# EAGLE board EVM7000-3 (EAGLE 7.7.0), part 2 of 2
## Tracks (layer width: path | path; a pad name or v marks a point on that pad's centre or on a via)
109
  Top 0.305: IC30.10 58.42,83.19 57.15,81.92 55.24,81.92 54.61,82.55 54.61,88.27 52.7,90.17 JP3.1
175  (via drill 0.5)
  Top 0.305: IC7.9 16.51,93.98 v16.51,78.11
  Bottom 0.305: v16.51,78.11 120.65,78.11 128.27,70.48 151.13,70.48 154.31,67.31 154.31,64.14 152.4,62.23 IC15.23
243  (via drill 0.5)
  Top 0.305: v36.2,130.81 v36.2,79.38
  Bottom 0.305: IC8.1 11.43,134.62 15.24,130.81 v36.2,130.81 | v36.2,79.38 36.83,78.74 121.28,78.74 128.91,71.12 151.76,71.12 154.94,67.94 154.94,62.23 152.4,59.69 IC15.22
6522  (via drill 0.5)
  Top 0.305: v41.27,80.01 41.27,90.17 v42.55,91.44
  Bottom 0.305: v42.55,91.44 IC34.23 | IC15.21 152.4,57.15 155.57,60.33 155.57,68.58 152.4,71.75 129.54,71.75 121.92,79.38 41.91,79.38 v41.27,80.01
!ENABLE  (via drill 0.5)
  Top 0.305: IC1.16 37.47,59.69 35.56,57.78 35.56,46.35 v37.47,44.45 | IC29.19 69.22,44.45 67.31,42.55 v67.31,38.1
  Bottom 0.305: v37.47,44.45 46.99,44.45 48.26,45.72 52.7,45.72 60.33,38.1 v67.31,38.1 67.94,38.1 73.03,33.02 88.9,33.02 90.17,31.75 IC33.3
+12V  (3 unrouted)
  Bottom 1.27: 133.35,9.53 X1.4 132.72,17.78 C26.+ | 154.31,9.53 VR1.1 | 149.22,9.53 144.78,13.34 | P3.3 161.29,35.56 158.12,32.38 151.76,32.38 149.86,30.48 149.86,24.77 C27.1 142.24,17.14 142.24,13.34
  Bottom 2.54: 133.35,9.53 137.16,9.53 137.16,9.87 J3.2 137.79,10.16 140.81,13.18 144.94,13.18 149.22,9.53 154.31,9.53
/LA  (via drill 0.5)
  Top 0.305: IC33.17 101.6,19.05 103.5,20.95 103.5,80.64 v101.6,82.55
  Bottom 0.305: IC30.4 66.04,90.81 68.58,88.27 73.03,88.27 76.2,85.09 99.06,85.09 v101.6,82.55
A0  (via drill 0.5)
  Top 0.305: IC21.12 93.98,44.45 97.16,47.62 97.16,78.74 98.42,80.01 v98.42,81.92 | IC34.37 47.62,127 44.45,123.83 44.45,83.19 43.81,82.55 v43.81,81.28
  Bottom 0.305: IC15.10 142.88,41.91 141.6,43.18 133.35,43.18 132.08,44.45 IC43.10 123.83,44.45 122.56,43.18 114.3,43.18 113.03,44.45 IC40.12 IC21.12 | v43.81,81.28 44.45,80.64 95.25,80.64 96.52,81.92 v98.42,81.92
A1  (via drill 0.5)
  Top 0.305: IC21.13 93.98,46.99 96.52,49.53 96.52,80.01 v97.16,80.64 | IC34.38 47.62,129.54 43.81,125.73 43.81,83.82 42.55,82.55 v42.55,80.64
  Bottom 0.305: IC15.9 142.88,44.45 141.6,45.72 133.35,45.72 132.08,46.99 IC43.9 123.83,46.99 122.56,45.72 114.94,45.72 113.67,46.99 IC40.11 IC21.13 | v42.55,80.64 43.18,80.01 96.52,80.01 v97.16,80.64
A2  (via drill 0.5)
  Top 0.305: IC21.14 93.98,49.53 95.89,51.44 v95.89,83.19 | IC34.36 47.62,124.46 45.09,121.92 v45.09,81.92
  Bottom 0.305: IC15.8 142.88,46.99 141.6,48.26 133.35,48.26 132.08,49.53 IC43.8 123.83,49.53 122.56,48.26 114.3,48.26 113.03,49.53 IC40.10 IC21.14 | v45.09,81.92 45.72,81.28 94.61,81.28 95.89,82.55 v95.89,83.19
A3  (via drill 0.5)
  Top 0.305: IC21.15 93.98,52.07 95.25,53.34 95.25,81.28 v93.98,82.55 | IC34.35 47.62,121.92 45.72,120.02 45.72,83.19 v46.35,82.55
  Bottom 0.305: IC15.7 142.88,49.53 141.6,50.8 133.35,50.8 132.08,52.07 IC43.7 123.83,52.07 122.56,50.8 114.3,50.8 113.03,52.07 IC40.9 IC21.15 | v46.35,82.55 46.99,81.92 93.34,81.92 v93.98,82.55
A4
  Bottom 0.305: IC15.6 142.88,52.07 141.6,53.34 133.35,53.34 132.08,54.61 IC43.6 123.83,54.61 122.56,53.34 114.3,53.34 113.03,54.61 IC40.8 IC21.16
A5
  Bottom 0.305: IC15.5 142.88,54.61 141.6,55.88 133.35,55.88 132.08,57.15 IC43.5 123.83,57.15 122.56,55.88 114.3,55.88 113.03,57.15 IC40.7 IC21.17
A6
  Bottom 0.305: IC15.4 142.88,57.15 141.6,58.42 133.35,58.42 132.08,59.69 IC43.4 123.83,59.69 122.56,58.42 114.3,58.42 113.03,59.69 IC40.6 IC21.18
A7
  Bottom 0.305: IC15.2 142.88,62.23 141.6,60.96 133.35,60.96 132.08,62.23 IC43.3 123.83,62.23 122.56,60.96 114.3,60.96 113.03,62.23 IC40.5 IC21.19
A8  (via drill 0.5)
  Top 0.305: IC40.27 120.02,59.69 117.47,57.15 117.47,31.11 v116.84,30.48
  Bottom 0.305: IC13.18 88.9,31.75 90.17,30.48 v116.84,30.48 | IC40.27 122.56,59.69 123.83,60.96 132.08,60.96 133.35,59.69 IC43.25 IC15.3
A9  (via drill 0.5)
  Top 0.305: v117.47,25.4 118.11,26.04 118.11,55.24 120.02,57.15 IC40.26
  Bottom 0.305: IC13.17 88.27,29.21 90.81,26.67 IC33.5 96.52,26.67 97.79,25.4 v117.47,25.4 | IC40.26 122.56,57.15 123.83,58.42 132.08,58.42 133.35,57.15 IC43.24
A10  (via drill 0.5)
  Top 0.305: v119.38,22.86 119.38,48.9 120.02,49.53 IC40.23
  Bottom 0.305: IC13.16 88.27,26.67 90.81,24.13 IC33.6 96.52,24.13 97.79,22.86 v119.38,22.86 | IC40.23 122.56,49.53 123.83,50.8 132.08,50.8 133.35,49.53 IC43.21
A11  (via drill 0.5)
  Top 0.305: v118.11,20.32 118.11,23.5 118.75,24.13 118.75,53.34 120.02,54.61 IC40.25
  Bottom 0.305: IC13.15 88.27,24.13 90.81,21.59 IC33.7 96.52,21.59 97.79,20.32 v118.11,20.32 | IC40.25 122.56,54.61 123.83,55.88 132.08,55.88 133.35,54.61 IC43.23
A12  (via drill 0.5)
  Top 0.305: v118.11,17.78 127,26.67 127,63.5 125.73,64.77 IC43.2
  Bottom 0.305: IC13.14 88.27,21.59 90.81,19.05 IC33.8 96.52,19.05 97.79,17.78 v118.11,17.78 | IC40.4 113.03,64.77 114.3,63.5 122.56,63.5 123.83,64.77 IC43.2
A13  (via drill 0.5)
  Top 0.305: v118.11,15.24 128.27,25.4 v128.27,63.5
  Bottom 0.305: IC13.13 88.27,19.05 90.81,16.51 IC33.9 96.52,16.51 97.79,15.24 v118.11,15.24 | IC40.28 122.56,62.23 123.83,63.5 v128.27,63.5 132.08,63.5 133.35,62.23 IC43.26
A14  (via drill 0.5)
  Top 0.305: v115.57,10.16 129.54,24.13 v129.54,69.22
  Bottom 0.305: IC13.11 88.27,13.97 90.81,11.43 IC33.11 96.52,11.43 97.79,10.16 v115.57,10.16 | IC40.3 113.03,67.31 114.3,68.58 128.91,68.58 v129.54,69.22 130.18,68.58 141.6,68.58 142.24,67.94 142.24,66.04 140.97,64.77 IC43.27
A15  (via drill 0.5)
  Top 0.305: v115.57,12.7 115.57,32.38 116.84,33.66 116.84,66.04 120.65,69.85 IC40.31
  Bottom 0.305: IC13.12 88.27,16.51 90.81,13.97 IC33.10 96.52,13.97 97.79,12.7 v115.57,12.7
AD0
  Bottom 0.305: IC12.28 65.41,41.91 69.22,46.99 IC29.18 73.03,46.99 74.3,45.72 80.01,45.72 81.28,44.45 IC21.9
AD1
  Bottom 0.305: IC12.29 65.41,44.45 69.22,49.53 IC29.17 73.03,49.53 74.3,48.26 80.01,48.26 81.28,46.99 IC21.8
AD2
  Bottom 0.305: IC12.30 65.41,46.99 69.22,52.07 IC29.16 73.03,52.07 74.3,50.8 80.01,50.8 81.28,49.53 IC21.7
AD3
  Bottom 0.305: IC12.31 65.41,49.53 69.22,54.61 IC29.15 73.03,54.61 74.3,53.34 80.01,53.34 81.28,52.07 IC21.6
AD4
  Bottom 0.305: IC12.32 65.41,52.07 69.22,57.15 IC29.14 73.03,57.15 74.3,55.88 80.01,55.88 81.28,54.61 IC21.5
AD5
  Bottom 0.305: IC12.33 65.41,54.61 69.22,59.69 IC29.13 73.03,59.69 74.3,58.42 80.64,58.42 81.92,57.15 IC21.4
AD6
  Bottom 0.305: IC12.34 65.41,57.15 69.22,62.23 IC29.12 73.03,62.23 74.3,60.96 80.64,60.96 81.92,59.69 IC21.3
AD7
  Bottom 0.305: IC12.35 65.41,59.69 69.22,64.77 IC29.11 73.03,64.77 74.3,63.5 80.64,63.5 81.92,62.23 IC21.2
CLK  (via drill 0.5)
  Top 0.305: IC30.12 63.5,76.2 v60.33,73.03
  Bottom 0.305: IC30.12 63.5,83.19 | IC1.12 39.37,69.85 43.18,73.66 59.69,73.66 v60.33,73.03
D0  (via drill 0.5)
  Top 0.305: IC29.2 78.11,44.45 83.82,50.16 v83.82,115.57 83.19,116.2 83.19,138.43 84.45,139.7 IC9.2 85.72,139.7 88.27,142.24 IC10.18
  Bottom 0.305: IC43.11 123.83,41.91 122.56,40.64 114.3,40.64 113.03,41.91 IC40.13 96.52,41.91 95.25,43.18 81.28,43.18 80.01,44.45 IC29.2 | IC24.3 IC28.18 94.61,114.3 93.34,115.57 v83.82,115.57 82.55,115.57 81.28,116.84 IC26.2 75.56,116.84 74.3,115.57 69.85,115.57 68.58,116.84 IC25.2 64.14,116.84 62.87,115.57 57.78,115.57 56.52,116.84 IC27.2 IC34.33
D1  (via drill 0.5)
  Top 0.305: IC29.3 78.11,46.99 83.19,52.07 83.19,112.71 v82.87,113.03 82.55,113.35 82.55,140.34 84.45,142.24 IC9.3 85.72,142.24 88.27,144.78 IC10.17 | v107.95,45.72 107.95,40.64 106.68,39.37 IC40.14
  Bottom 0.305: IC40.14 113.03,39.37 114.3,38.1 122.56,38.1 123.83,39.37 IC43.12 | IC24.18 108.58,114.3 107.31,113.03 101.6,113.03 100.33,111.76 IC28.17 94.61,111.76 93.34,113.03 v82.87,113.03 82.55,113.03 81.28,114.3 IC26.3 75.56,114.3 74.3,113.03 69.85,113.03 68.58,114.3 IC25.3 64.14,114.3 62.87,113.03 57.78,113.03 56.52,114.3 IC27.3 IC34.32 | IC29.3 80.01,46.99 81.28,45.72 v107.95,45.72
D2  (via drill 0.5)
  Top 0.305: IC29.4 78.11,49.53 82.55,53.98 82.55,110.81 v82.23,111.12 81.92,111.44 81.92,142.24 84.45,144.78 IC9.4 85.72,144.78 88.27,147.32 IC10.16 | v108.58,48.26 109.22,47.62 109.22,39.37 106.68,36.83 IC40.15
  Bottom 0.305: IC40.15 113.03,36.83 114.3,35.56 122.56,35.56 123.83,36.83 IC43.13 | IC24.4 102.23,111.76 99.69,109.22 IC28.16 94.61,109.22 93.34,110.49 82.87,110.49 v82.23,111.12 81.6,111.76 IC26.4 75.56,111.76 74.3,110.49 69.85,110.49 68.58,111.76 IC25.4 64.14,111.76 62.87,110.49 57.78,110.49 56.52,111.76 IC27.4 IC34.31 | IC29.4 80.01,49.53 81.28,48.26 v108.58,48.26
D3  (via drill 0.5)
  Top 0.305: IC29.5 78.11,52.07 81.92,55.88 81.92,108.9 v81.6,109.22 81.28,109.54 81.28,144.15 84.45,147.32 IC9.5 85.72,147.32 88.27,149.86 IC10.15 | v109.22,50.8 109.86,50.16 v109.86,35.56
  Bottom 0.305: IC24.17 108.58,111.76 107.31,110.49 102.87,110.49 99.06,106.68 IC28.15 94.61,106.68 93.34,107.95 82.87,107.95 v81.6,109.22 IC26.5 75.56,109.22 74.3,107.95 69.85,107.95 68.58,109.22 IC25.5 64.14,109.22 62.87,107.95 57.78,107.95 56.52,109.22 IC27.5 IC34.30 | IC29.5 80.01,52.07 81.28,50.8 v109.22,50.8 | v109.86,35.56 113.03,35.56 114.3,34.29 IC40.17 122.56,34.29 123.83,35.56 132.08,35.56 133.35,34.29 IC43.15
D4  (via drill 0.5)
  Top 0.305: IC29.6 78.11,54.61 81.28,57.78 81.28,106.36 v80.96,106.68 80.64,107 80.64,146.05 84.45,149.86 IC9.6 85.72,149.86 88.27,152.4 IC10.14 | v109.86,53.34 110.49,52.7 110.49,38.73 v111.12,38.1
  Bottom 0.305: IC43.16 133.35,36.83 132.08,38.1 123.83,38.1 122.56,36.83 IC40.18 114.3,36.83 113.03,38.1 v111.12,38.1 | IC24.7 IC28.14 95.25,104.14 93.98,105.41 82.55,105.41 81.28,106.68 v80.96,106.68 IC26.6 75.56,106.68 74.3,105.41 69.85,105.41 68.58,106.68 IC25.6 64.14,106.68 62.87,105.41 57.78,105.41 56.52,106.68 IC27.6 IC34.29 41.27,106.68 40.01,105.41 19.05,105.41 | IC29.6 80.01,54.61 81.28,53.34 v109.86,53.34 | IC7.4 12.7,104.14 13.97,105.41 19.05,105.41 | IC8.11 17.78,127 19.05,125.73 19.05,105.41
D5  (via drill 0.5)
  Top 0.305: IC29.7 78.11,57.15 80.64,59.69 80.64,102.23 78.74,104.14 | v110.49,55.88 111.12,55.24 111.12,41.27 v111.76,40.64 | IC26.7 78.74,104.14 | 78.74,104.14 80.01,105.41 80.01,147.96 84.45,152.4 IC9.7 85.72,152.4 88.27,154.94 IC10.13 | IC8.8 17.78,119.38 19.05,118.11 19.05,105.41 17.78,104.14 IC7.13
  Bottom 0.305: IC43.17 133.35,39.37 132.08,40.64 123.83,40.64 122.56,39.37 IC40.19 114.3,39.37 113.03,40.64 v111.76,40.64 | IC24.14 108.58,104.14 107.31,102.87 101.6,102.87 100.33,101.6 IC28.13 94.61,101.6 93.34,102.87 82.55,102.87 81.28,104.14 IC26.7 75.56,104.14 74.3,102.87 69.85,102.87 68.58,104.14 IC25.7 64.14,104.14 62.87,102.87 57.78,102.87 56.52,104.14 IC27.7 IC34.28 41.27,104.14 40.01,102.87 31.11,102.87 29.84,104.14 IC7.13 | IC29.7 80.64,57.15 81.92,55.88 v110.49,55.88
D6  (via drill 0.5)
  Top 0.305: IC29.8 78.11,59.69 80.01,61.59 80.01,100.33 78.74,101.6 IC26.8 77.47,101.6 76.2,102.87 76.2,120.02 79.38,123.19 79.38,149.86 84.45,154.94 IC9.8 85.72,154.94 88.27,157.48 IC10.12 | v111.12,58.42 111.76,57.78 111.76,43.81 v112.39,43.18 | IC8.10 17.78,124.46 20.32,121.92 20.32,102.23 v19.68,101.6
  Bottom 0.305: IC43.18 133.35,41.91 132.08,43.18 123.83,43.18 122.56,41.91 IC40.20 114.3,41.91 113.03,43.18 v112.39,43.18 | IC24.8 102.23,101.6 99.69,99.06 IC28.12 94.61,99.06 93.34,100.33 82.55,100.33 81.28,101.6 IC26.8 75.56,101.6 74.3,100.33 69.85,100.33 68.58,101.6 IC25.8 64.14,101.6 62.87,100.33 57.78,100.33 56.52,101.6 IC27.8 IC34.27 41.27,101.6 40.01,100.33 31.11,100.33 28.57,102.87 19.68,102.87 | IC29.8 80.64,59.69 81.92,58.42 v111.12,58.42 | 19.68,102.87 13.97,102.87 12.7,101.6 IC7.5 | 19.68,102.87 v19.68,101.6
D7  (via drill 0.5)
  Top 0.305: IC29.9 78.11,62.23 79.38,63.5 79.38,91.44 76.2,94.61 76.2,97.79 77.47,99.06 | 77.47,99.06 IC26.9 | v111.76,60.96 112.39,60.33 112.39,46.35 v113.03,45.72 | 77.47,99.06 75.56,100.97 75.56,120.65 78.74,123.83 78.74,132.72 75.56,135.89 75.56,150.5 76.2,151.13 78.74,151.13 83.82,156.21 83.82,156.84 84.45,157.48 IC9.9 85.72,157.48 88.27,160.02 IC10.11 | IC8.9 17.78,121.92 19.68,120.02 19.68,103.5 17.78,101.6 IC7.12
  Bottom 0.305: IC43.19 133.35,44.45 132.08,45.72 123.83,45.72 122.56,44.45 IC40.21 114.3,44.45 v113.03,45.72 | IC24.13 108.58,101.6 107.31,100.33 102.87,100.33 99.06,96.52 IC28.11 94.61,96.52 93.34,97.79 82.55,97.79 81.28,99.06 IC26.9 75.56,99.06 74.3,97.79 69.85,97.79 68.58,99.06 IC25.9 64.14,99.06 62.87,97.79 57.78,97.79 56.52,99.06 IC27.9 IC34.26 41.27,99.06 40.01,97.79 21.59,97.79 17.78,101.6 IC7.12 | IC29.9 80.64,62.23 81.92,60.96 v111.76,60.96
DSR1  (via drill 0.5)
  Top 0.305: IC2.9 69.85,157.48 68.58,156.21 v68.58,148.59 | R44.2 57.78,152.4 52.7,147.32 P5.2
  Bottom 0.305: v68.58,148.59 57.15,148.59 55.88,147.32 P5.2
DSR2
  Top 0.305: R43.2 38.73,149.86 41.27,147.32 P4.2
  Bottom 0.305: IC2.18 62.87,142.24 61.59,143.51 46.35,143.51 42.55,147.32 P4.2
DTR1
  Bottom 0.305: IC2.15 P5.3
DTR2
  Bottom 0.305: IC2.6 67.94,149.86 66.67,151.13 43.81,151.13 42.55,149.86 P4.3
GAL2
  Bottom 0.305: IC33.19 134.62,24.13 140.97,30.48 143.51,30.48 146.69,33.66 146.69,37.47 144.78,39.37 IC15.11
GND  (via drill 0.5)  (1 unrouted)
  Top 0.305: IC27.1 53.98,119.38 55.24,118.11 55.24,97.79 53.98,96.52 IC27.10 | C5.2 87.63,38.73 87.63,35.56 86.36,34.29 IC13.19 | IC30.13 66.04,73.66 IC12.40 | v132.08,95.25 132.08,103.5 136.53,107.95 IC19.20 | IC9.1 85.72,137.16 87,138.43 90.17,138.43 90.81,139.06 90.81,160.66 90.17,161.29 87,161.29 85.72,160.02 IC9.10
  Top 1.27: JP1.1 C10.2 76.2,65.41 | 76.2,65.41 76.83,64.77 IC29.10 | 76.2,65.41 76.2,64.77 74.93,63.5 74.93,40.64 C18.2 | 87,65.41 C7.2 88.27,69.85 88.27,92.08 90.17,93.98 IC28.10 | 87,65.41 86.36,64.77 IC21.1 | 87,65.41 87,64.77 88.27,63.5 88.27,43.18 87,41.91 | 87,41.91 IC21.10 | 87,41.91 C5.2 | IC13.1 79.38,36.83 80.64,35.56 80.64,15.24 79.38,13.97 | 79.38,13.97 IC13.10 | 79.38,13.97 C8.2 | IC33.12 93.98,8.89 94.61,8.26 | 94.61,8.26 C6.2 | C11.2 95.89,9.53 94.61,8.26 | C2.2 114.94,71.75 114.94,36.83 111.76,33.66 106.68,33.66 IC40.16 C25.2 | C9.2 44.45,73.03 | 44.45,73.03 45.09,72.39 IC1.10 | 12.06,119.38 12.06,137.16 C16.2 | 12.06,119.38 12.06,115.57 | 12.06,115.57 12.06,93.98 | 12.06,93.98 12.06,91.44 C13.- | IC7.8 12.06,93.98 | C20.2 12.06,115.57 | IC8.7 12.06,119.38 | 44.45,73.03 43.18,71.75 v43.18,52.07 43.18,49.53 | 43.18,49.53 IC1.1 | 43.18,49.53 43.18,42.55 42.55,41.91 C12.2 42.55,26.04 | 42.55,26.04 C43.- | 42.55,26.04 SW1.1 SW1.2 | C1.2 54.61,63.5 63.5,72.39 IC12.40 | C21.2 146.69,66.04 146.69,36.83 | 146.69,36.83 146.69,35.56 | 146.69,35.56 C22.2 | 146.69,36.83 IC15.12 144.15,35.56 C22.2 | QG2.7 45.09,10.79 C24.2 | C27.2 145.41,27.94 | 145.41,27.94 142.24,27.94 C14.- 142.88,22.23 142.88,19.05 145.41,16.51 145.41,10.16 142.24,6.99 | C22.2 145.41,27.94 | 146.69,35.56 151.13,31.11 151.13,18.41 157.48,12.06 VR1.2
  Bottom 0.305: IC27.1 56.52,119.38 57.78,118.11 62.87,118.11 64.14,119.38 IC25.1 68.58,119.38 69.85,118.11 74.3,118.11 75.56,119.38 IC26.1 | IC1.19 v43.18,52.07 | IC19.14 122.56,95.25 123.19,95.89 126.36,95.89 127,95.25 v132.08,95.25 | 147.32,147.32 IC3.3 | IC3.5 152.4,147.32
  Bottom 1.27: IC27.10 53.34,94.61 55.88,94.61 | 55.88,94.61 65.41,94.61 | 65.41,94.61 IC25.10 | 65.41,94.61 78.11,94.61 | 78.11,94.61 IC26.10 | 78.11,94.61 90.17,94.61 | 90.17,94.61 IC28.10 | 90.17,94.61 104.14,94.61 | 104.14,94.61 IC24.10 | C18.2 78.11,39.37 | 78.11,39.37 C5.2 | 78.11,39.37 IC13.1 | IC40.16 107.95,32.38 125.09,32.38 | 125.09,32.38 142.24,32.38 144.15,34.29 | 144.15,34.29 IC15.12 | IC43.14 125.09,32.38 | JP1.1 76.2,73.03 74.93,74.3 66.67,74.3 IC12.40 62.23,74.93 C9.2 43.18,74.93 41.27,76.83 37.47,76.83 J8.40 30.48,74.93 16.51,74.93 8.89,67.31 C3.- 3.17,66.04 | IC29.10 IC21.1 | IC30.8 55.88,94.61 | 104.14,94.61 120.65,94.61 121.28,95.25 IC19.14 | 85.09,161.93 94.61,161.93 IC10.10 100.33,160.02 | 85.09,161.93 IC9.10 | 85.09,161.93 71.12,161.93 IC2.10 | 100.33,160.02 109.86,160.02 | C10.2 C7.2 88.9,70.48 100.33,70.48 105.41,75.56 C2.2 | 109.86,160.02 C23.2 109.86,153.03 110.49,152.4 IC11.7 | C17.2 33.66,134.62 IC34.1 21.59,134.62 19.05,132.08 IC8.13 16.51,132.08 10.79,137.79 C16.2 3.17,138.43 | C19.2 100.33,160.02 | SW1.2 49.53,19.05 | 49.53,19.05 53.98,19.05 C1.2 | QG2.7 49.53,19.05 | 11.43,164.47 12.06,164.47 | C13.- 3.17,88.9 | 144.15,34.29 C22.2 | C6.2 94.61,3.17 | C8.2 79.38,3.17 | P7.1 73.66,3.17 | 170.81,128.27 IC20.40 163.19,128.91 C30.2 163.19,147.32 | 170.81,128.27 177.8,128.27 | 177.8,128.27 192.41,128.27 | C25.2 106.05,3.17 | C24.2 45.09,3.17 | 134.62,164.47 134.62,160.66 | 134.62,160.66 134.62,146.05 | 134.62,146.05 JP2.3 | 109.86,160.02 109.86,164.47 | 36.83,164.47 36.83,158.12 37.47,157.48 P4.6 P5.6 | 134.62,146.05 C15.2 140.34,147.32 147.32,147.32 152.4,147.32 160.02,147.32 | 160.02,147.32 IC3.8 | 160.02,147.32 163.19,147.32
  Bottom 1.27: 163.19,147.32 180.34,147.32 181.61,146.05 IC4.7 192.41,144.78 | C29.2 170.81,128.27 | C28.- 177.8,128.27 | C14.- 135.89,21.59 131.44,21.59 128.91,19.05 128.91,18.41 | 128.91,18.41 128.91,9.53 | 128.91,18.41 C26.- | C4.- 134.62,160.66 | R16.2 25.4,164.47 | VR1.2 157.48,20.95
  Bottom 2.54: 12.06,164.47 25.4,164.47 36.83,164.47 109.86,164.47 134.62,164.47 179.07,164.47 192.41,151.13 192.41,144.78 192.41,128.27 192.41,46.35 | 192.41,46.35 192.41,27.3 | 192.41,27.3 192.41,8.26 | 192.41,8.26 192.41,4.45 191.13,3.17 179.07,3.17 | 179.07,3.17 157.48,3.17 | 157.48,3.17 142.24,3.17 | 142.24,3.17 128.91,3.17 | 128.91,3.17 106.05,3.17 94.61,3.17 79.38,3.17 73.66,3.17 45.09,3.17 26.04,3.17 3.17,26.04 3.17,66.04 3.17,88.9 3.17,138.43 3.17,157.48 10.16,164.47 11.43,164.47 | 179.07,3.17 179.07,8.26 | 179.07,8.26 179.07,27.3 | 179.07,27.3 SX21.1 192.41,27.3 | 179.07,27.3 SX21.2 | 179.07,27.3 179.07,46.35 | 179.07,46.35 SX12.1 192.41,46.35 | 179.07,46.35 SX12.2 | 179.07,8.26 SX5.1 192.41,8.26 | 179.07,8.26 SX5.2 | X1.2 128.91,9.53 | 128.91,9.53 X1.3 | 128.91,9.53 128.91,3.17 | 142.24,3.17 142.24,7.08 | VR1.2 157.48,3.17
IC24  (via drill 0.5)
  Top 0.305: IC24.11 v111.76,80.64
  Bottom 0.305: v111.76,80.64 121.92,80.64 130.18,72.39 153.03,72.39 156.21,69.22 156.21,58.42 152.4,54.61 IC15.20
IC25  (via drill 0.5)
  Top 0.305: IC25.11 77.47,92.08 v77.47,87.63
  Bottom 0.305: v77.47,87.63 78.74,86.36 121.28,86.36 132.72,74.93 155.57,74.93 158.75,71.75 158.75,50.8 152.4,44.45 IC15.16
IC26  (via drill 0.5)
  Top 0.305: IC26.11 84.45,95.25 84.45,88.27 v85.09,87.63
  Bottom 0.305: v85.09,87.63 85.72,87 121.92,87 133.35,75.56 156.21,75.56 159.38,72.39 159.38,48.9 152.4,41.91 IC15.15
IC27  (via drill 0.5)
  Top 0.305: IC27.11 62.87,96.52 64.14,97.79 69.22,97.79 71.75,95.25 73.03,95.25 76.2,92.08 v76.2,87
  Bottom 0.305: v76.2,87 77.47,85.72 120.65,85.72 132.08,74.3 154.94,74.3 158.12,71.12 158.12,52.7 152.4,46.99 IC15.17
IC28  (via drill 0.5)
  Top 0.305: IC28.1 88.9,119.38 87.63,118.11 87.63,95.89 85.41,93.66 v85.41,89.22
  Bottom 0.305: v85.41,89.22 87,87.63 122.56,87.63 133.99,76.2 156.84,76.2 160.02,73.03 160.02,46.99 152.4,39.37 IC15.14 | IC28.1 92.71,119.38 95.25,116.84 IC28.19
INT1
  Bottom 0.305: IC12.13 48.26,41.91 46.99,40.64 26.04,40.64 24.77,41.91 J8.13
INT3
  Bottom 0.305: J8.12 24.77,44.45 26.04,43.18 46.99,43.18 48.26,44.45 IC12.12
LATCH  (via drill 0.5)
  Top 0.305: IC1.17 37.47,57.15 36.2,55.88 36.2,48.26 v37.47,46.99 | IC33.2 92.71,34.29 91.44,35.56 91.44,37.47 92.08,38.1 92.71,38.1 93.34,38.73 IC21.11
  Bottom 0.305: IC21.11 88.9,41.91 87.63,40.64 60.33,40.64 52.7,48.26 48.26,48.26 46.99,46.99 v37.47,46.99
N$1
  Bottom 0.305: IC12.1 48.9,72.39 46.35,69.85 IC1.9
N$2
  Bottom 0.305: IC12.2 48.9,69.85 46.35,67.31 IC1.8
N$3
  Bottom 0.305: IC12.3 48.9,67.31 46.35,64.77 IC1.7
N$4
  Top 0.305: SW1.3 SW1.4
  Bottom 0.61: R39.2 38.1,26.04 SW1.3
N$5
  Bottom 0.305: IC12.4 48.9,64.77 46.35,62.23 IC1.6
N$6
  Bottom 0.305: IC12.19 55.24,26.67 59.05,22.86 68.58,22.86 72.39,19.05 IC13.8
N$7
  Bottom 0.305: IC12.20 55.88,24.13 57.78,22.23 67.31,22.23 73.03,16.51 IC13.9
N$8
  Bottom 0.305: IC12.5 48.9,62.23 46.35,59.69 IC1.5
N$9
  Bottom 0.305: IC1.4 46.99,57.15 48.26,58.42 51.44,58.42 62.87,69.85 IC12.39
N$10
  Bottom 0.305: IC12.27 67.94,39.37 73.03,34.29 IC13.2
N$11
  Bottom 0.305: IC13.3 73.03,31.75 67.94,36.83 IC12.26
N$12
  Bottom 0.305: IC12.24 69.85,31.75 72.39,29.21 IC13.4
N$13
  Bottom 0.305: IC1.3 46.99,54.61 48.26,55.88 51.44,55.88 62.87,67.31 IC12.38
N$14
  Top 1.27: P1.1 C12.1
  Bottom 1.27: P1.1 J8.25
N$15
  Bottom 0.305: IC12.37 62.87,64.77 51.44,53.34 48.26,53.34 46.99,52.07 IC1.2
N$16
  Bottom 0.61: R13.2 EXTRA.K
N$17
  Bottom 0.305: IC13.5 71.75,26.67 69.22,29.21 IC12.23
N$18
  Bottom 0.305: IC12.22 69.22,26.67 71.75,24.13 IC13.6
N$19
  Bottom 0.305: IC12.21 69.22,24.13 71.75,21.59 IC13.7
N$20
  Bottom 0.61: IC11.4 119.38,144.78 R13.1
N$21
  Bottom 0.305: P8.1 IC34.40
N$22
  Bottom 0.305: IC34.39 P8.2
N$23  (via drill 0.5)
  Top 0.305: IC20.17 147.96,87.63 136.53,76.2 136.53,29.21 v120.65,13.34
  Bottom 0.305: P7.2 74.3,11.43 75.56,12.7 86.36,12.7 91.44,7.62 114.94,7.62 v120.65,13.34
N$24
  Bottom 0.305: IC34.18 P9.1
N$25
  Bottom 0.305: P9.2 IC34.19
N$26  (via drill 0.5)
  Top 0.305: v73.03,143.51 73.03,153.67 71.75,154.94 IC2.8
  Bottom 0.305: IC10.5 93.34,147.32 92.08,146.05 81.92,146.05 80.64,147.32 IC9.16 76.83,147.32 v73.03,143.51 67.94,143.51 66.67,144.78 IC2.17
N$27
  Top 0.305: IC2.11 64.14,160.02 65.41,158.75 65.41,144.78 70.48,139.7 IC2.2
  Bottom 0.305: IC10.3 93.34,142.24 92.08,140.97 81.92,140.97 80.64,142.24 IC9.18 76.2,142.24 73.66,139.7 IC2.2
N$28
  Bottom 0.305: IC10.7 93.34,152.4 92.08,151.13 76.2,151.13 72.39,147.32 IC2.5 IC2.16
N$29
  Bottom 0.305: IC10.8 93.34,154.94 92.08,153.67 73.66,153.67 72.39,152.4 IC2.7 IC2.14
N$30
  Bottom 0.305: IC10.2 93.34,139.7 92.08,138.43 81.92,138.43 80.64,139.7 IC9.19 76.2,139.7 73.66,137.16 IC2.1 68.58,137.16 66.04,139.7 IC2.19
N$31
  Bottom 0.305: IC9.17 80.64,144.78 81.92,143.51 92.08,143.51 93.34,144.78 IC10.4 97.16,144.78 99.69,147.32 100.97,147.32 102.23,146.05 106.05,146.05 107.31,144.78 107.31,137.79 109.22,135.89 125.09,135.89 132.08,143.51 JP2.2
N$32
  Bottom 0.305: IC9.15 80.64,149.86 81.92,148.59 92.08,148.59 93.34,149.86 IC10.6
N$33
  Bottom 0.305: JP4.2 147.32,159.38 149.22,161.29 172.72,161.29 179.07,154.94 IC4.9
N$34
  Bottom 0.305: JP5.2 157.48,159.38 158.75,160.66 172.09,160.66 173.99,158.75 IC4.11
N$36
  Top 0.61: Q1.E 184.15,56.52 184.15,42.93 SX21.4
  Bottom 0.406: Q1.E R5.1
N$37
  Bottom 0.406: Q2.E R4.1
  Bottom 0.61: Q2.E 187.32,58.8 SX12.4
N$38
  Bottom 0.406: R6.1 R5.2 Q1.B
N$39
  Top 0.305: R7.2 183.51,149.86 181.61,151.76 IC4.8
N$40
  Bottom 0.406: R7.1 R4.2 Q2.B
N$41  (via drill 0.7)
  Top 0.61: v127,135.25 127.64,135.25 132.08,139.7 132.08,140.97 131.44,141.6 126.36,141.6 D4.2
  Top 1.27: IC19.1 121.92,130.18 v127,135.25 | D2.2 C28.+
  Bottom 0.61: IC11.2 120.65,139.7 D4.2 | D3.2 D2.2 D1.2 R3.2
  Bottom 1.27: v127,135.25 146.05,135.25 162.56,118.11 IC20.36 C29.1 C28.+
N$42
  Top 0.305: R6.2 173.99,129.54 172.09,131.44 172.09,140.34 175.26,143.51 175.26,147.96 176.53,149.22 IC4.10
N$43
  Bottom 0.406: R9.2 R8.2 Q3.B
N$44
  Bottom 0.61: D1.1 Q2.C
N$45
  Top 0.305: IC4.12 171.45,149.22 170.18,147.96 170.18,133.99 166.37,130.18 166.37,92.08 168.91,89.53 168.91,74.93 R9.1
N$46
  Bottom 0.305: IC10.9 97.16,157.48 99.06,155.57 99.06,149.86 100.33,148.59 106.68,148.59 108.58,146.69 108.58,139.7 109.86,138.43 123.19,138.43 JP2.1 129.54,147.32 R15.1
N$47
  Bottom 0.61: D2.1 Q1.C
N$48
  Bottom 0.61: Q3.C 168.28,69.22 D3.1
N$49
  Top 0.61: Q3.E 170.18,62.87 175.26,57.78 175.26,32.77 SX5.4
  Bottom 0.406: Q3.E R8.1
N$50
  Bottom 0.61: SWAP.K R14.2
N$51
  Bottom 1.27: P3.2 158.75,38.1 160.02,39.37 164.47,39.37 | 164.47,39.37 168.91,39.37 SX21.3 | 164.47,39.37 164.47,53.98 168.28,57.78 168.53,57.78 SX12.3
N$52
  Bottom 0.406: 113.03,151.13 107.95,151.13
  Bottom 0.61: R14.1 113.03,151.13 | 107.95,151.13 106.68,152.4 IC11.8
N$53
  Bottom 1.27: PWR.K R16.1
N$54
  Top 0.305: JP4.1 144.78,158.12 147.32,155.57 IC3.14
  Bottom 0.305: JP4.1 144.78,158.12 146.05,156.84 158.75,156.84 160.02,158.12 JP5.3
N$55
  Top 0.305: JP4.3 IC3.13
  Bottom 0.305: JP4.3 JP5.1
N$56
  Bottom 0.61: PGM.K R11.2
N$57
  Bottom 0.61: DATA.K R12.2
N$58
  Bottom 0.61: R12.1 128.27,149.86 D4.1
N$59
  Bottom 0.305: IC12.36 65.41,62.23 67.31,64.14 67.31,66.67 70.48,69.85 73.03,69.85 73.66,70.48 JP1.2
N$60
  Bottom 0.61: IC11.6 111.76,149.86 113.67,147.96 117.47,147.96 R11.1
N$63
  Top 0.305: IC34.25 48.9,96.52 50.16,95.25 50.16,88.9 51.44,87.63 JP3.2
N$64
  Top 0.305: IC30.14 68.58,85.09 66.04,87.63 64.14,87.63 60.96,90.81 IC30.6
N$65
  Top 1.27: JP7.1 VR1.3
  Bottom 1.27: VR1.3 JP7.1
N$66
  Top 0.305: IC30.1 73.66,92.08 72.39,93.34 57.78,93.34 57.15,92.71 57.15,88.27 55.88,87 IC30.9
OSC
  Bottom 0.305: P2.3 44.45,12.7 QG2.8
PC0
  Top 0.305: IC34.10 32.38,111.76 26.67,106.05 26.67,47.62 32.38,41.91 J8.28
PC1
  Top 0.305: IC34.11 32.38,109.22 27.3,104.14 27.3,49.53 32.38,44.45 J8.29
PC2
  Top 0.305: IC34.12 32.38,106.68 27.94,102.23 27.94,51.44 32.38,46.99 J8.30
PC3
  Top 0.305: IC34.13 32.38,104.14 28.57,100.33 28.57,53.34 32.38,49.53 J8.31
PC4
  Top 0.305: IC34.14 32.38,101.6 29.21,98.42 29.21,55.24 32.38,52.07 J8.32
PC5
  Top 0.305: IC34.15 32.38,99.06 29.84,96.52 29.84,57.15 32.38,54.61 J8.33
PC6
  Top 0.305: IC34.16 32.38,96.52 30.48,94.61 30.48,59.05 32.38,57.15 J8.34
PC7
  Top 0.305: IC34.17 32.38,93.98 31.11,92.71 31.11,60.96 32.38,59.69 J8.35
PD0
  Top 0.305: J8.27 32.38,39.37 26.04,45.72 26.04,106.68 31.11,111.76 31.11,130.81 32.38,132.08 IC34.2
PD1  (via drill 0.5)
  Top 0.305: J8.26 32.38,36.83 25.4,43.81 25.4,107.31 29.84,111.76 v29.84,129.54
  Bottom 0.305: v29.84,129.54 IC34.3
PD2  (via drill 0.5)
  Top 0.305: J8.24 32.38,31.75 24.77,40.01 24.77,107.95 28.57,111.76 v28.57,127
  Bottom 0.305: IC34.4 v28.57,127
PD3  (via drill 0.5)
  Top 0.305: J8.23 32.38,29.21 24.13,38.1 24.13,108.58 27.3,111.76 v27.3,124.46
  Bottom 0.305: IC34.5 v27.3,124.46
PD4  (via drill 0.5)
  Top 0.305: J8.22 32.38,26.67 23.5,36.2 23.5,109.22 26.04,111.76 v26.04,121.92
  Bottom 0.305: IC34.6 v26.04,121.92
PD5  (via drill 0.5)
  Top 0.305: J8.21 32.38,24.13 22.86,34.29 22.86,109.86 24.77,111.76 v24.77,119.38
  Bottom 0.305: v24.77,119.38 IC34.7
PD6  (via drill 0.5)
  Top 0.305: J8.20 18.41,24.13 22.23,27.94 22.23,110.49 23.5,111.76 v23.5,116.84
  Bottom 0.305: IC34.8 v23.5,116.84
PD7  (via drill 0.5)
  Top 0.305: J8.19 18.41,26.67 21.59,29.84 21.59,111.12 22.23,111.76 v22.23,114.3
  Bottom 0.305: v22.23,114.3 IC34.9
PHI2  (via drill 0.5)
  Top 0.305: IC33.18 101.6,21.59 102.87,22.86 102.87,79.38 v100.97,81.28
  Bottom 0.305: JP3.3 52.7,85.09 53.98,86.36 73.66,86.36 75.56,84.45 97.79,84.45 v100.97,81.28
PW0  (via drill 0.5)
  Top 0.305: IC33.1 94.61,38.1 94.61,40.64 97.79,43.81 97.79,78.11 99.69,80.01 99.69,117.47 100.33,118.11 102.23,118.11 103.5,116.84 IC24.2 | v108.58,119.38 108.58,121.92 101.6,128.91 101.6,148.59 102.87,149.86 IC11.9
  Bottom 0.305: IC24.2 105.41,116.84 107.95,119.38 v108.58,119.38
PW1
  Top 0.305: IC24.19 112.39,116.84 113.67,118.11 113.67,134.62 IC11.1
  Bottom 0.305: IC11.1 124.46,137.16 130.81,143.51 130.81,146.05 131.44,146.69 132.72,146.69 133.35,146.05 133.35,142.88 133.99,142.24 147.96,142.24 149.86,144.15 IC3.4
PW2
  Bottom 0.305: IC24.5 107.31,109.22 108.58,110.49 113.03,110.49 114.3,111.76 135.25,111.76 136.53,113.03 IC19.22 142.24,113.03 143.51,111.76 149.86,111.76 150.5,112.39 150.5,116.84 149.22,118.11 IC20.5
PW3
  Top 0.305: IC24.16 112.39,109.22 114.3,111.12 114.3,139.7 111.76,142.24 IC11.3
PW4  (via drill 0.5)
  Top 0.305: v146.05,107.95 146.05,104.78 147.96,102.87 IC20.11 | v133.35,106.68 133.35,122.56 136.53,125.73 IC19.27
  Bottom 0.305: IC24.6 107.31,106.68 108.58,105.41 113.03,105.41 114.3,106.68 v133.35,106.68 142.24,106.68 143.51,107.95 v146.05,107.95
PW5  (via drill 0.5)
  Top 0.305: IC24.15 112.39,106.68 114.94,109.22 114.94,139.7 | 114.94,139.7 114.94,144.15 111.76,147.32 IC11.5 | 114.94,139.7 v130.18,139.7 | IC4.13 168.91,149.86 167.64,148.59 167.64,143.51 167,142.88 156.21,142.88 154.94,144.15 IC3.6
  Bottom 0.305: v130.18,139.7 150.5,139.7 154.94,144.15 IC3.6
PW6
  Top 0.305: R38.2 100.97,101.6 103.5,99.06 IC24.9
  Bottom 0.305: IC24.9 107.31,99.06 108.58,97.79 113.03,97.79 114.3,96.52 142.24,96.52 143.51,95.25 IC20.14
PW7
  Bottom 0.305: IC24.12 114.94,99.06 120.02,104.14 142.24,104.14 143.51,105.41 IC20.10
PX0  (via drill 0.5)
  Top 0.305: IC28.2 90.81,116.84 95.89,111.76 95.89,95.25 v98.11,93.03 | IC19.11 122.56,102.87 125.09,100.33 125.09,95.25 v125.73,94.61
  Bottom 0.305: IC26.19 IC28.2 | v98.11,93.03 98.42,92.71 121.92,92.71 123.83,94.61 v125.73,94.61 126.36,93.98 150.5,93.98 151.76,95.25 160.66,95.25 163.19,97.79 IC20.28
PX1  (via drill 0.5)
  Top 0.305: IC28.3 90.81,114.3 95.25,109.86 95.25,93.98 v96.52,92.71 | IC19.12 122.56,100.33 124.46,98.42 124.46,93.98 v125.09,93.34
  Bottom 0.305: IC28.3 IC26.18 | v96.52,92.71 97.16,92.08 122.56,92.08 123.83,93.34 v125.09,93.34 | IC19.12 128.91,100.33 130.18,99.06 155.57,99.06 156.84,100.33 IC20.29
PX2  (via drill 0.5)
  Top 0.305: IC28.4 90.81,111.76 94.61,107.95 94.61,92.71 v95.25,92.08 | IC19.13 122.56,97.79 123.83,96.52 123.83,92.71 v124.46,92.08 | IC20.30 163.19,102.87 161.29,100.97 v161.29,91.44
  Bottom 0.305: IC26.17 IC28.4 | v95.25,92.08 95.89,91.44 123.83,91.44 v124.46,92.08 125.73,92.08 126.36,92.71 146.05,92.71 147.32,91.44 v161.29,91.44
PX3  (via drill 0.5)
  Top 0.305: IC28.5 90.81,109.22 93.98,106.05 v93.98,91.44 | IC19.15 v137.16,91.44 | v160.02,88.9 160.02,102.23 163.19,105.41 IC20.31
  Bottom 0.305: IC28.5 IC26.16 | v93.98,91.44 94.61,90.81 126.36,90.81 127.64,92.08 136.53,92.08 v137.16,91.44 144.78,91.44 147.32,88.9 v160.02,88.9
PX4  (via drill 0.5)
  Top 0.305: IC28.6 90.81,106.68 93.34,104.14 93.34,92.71 92.71,92.08 v92.71,90.81 | IC19.16 136.53,97.79 135.25,96.52 135.25,91.44 v135.89,90.81 | v158.75,96.52 158.75,103.5 163.19,107.95 IC20.32
  Bottom 0.305: IC26.15 IC28.6 | v92.71,90.81 93.34,90.17 127,90.17 128.27,91.44 135.25,91.44 v135.89,90.81 | IC19.16 142.24,97.79 143.51,96.52 v158.75,96.52
PX5  (via drill 0.5)
  Top 0.305: IC28.7 90.81,104.14 92.71,102.23 92.71,93.34 91.44,92.08 v91.44,90.17 | v134.62,90.17 134.62,98.42 136.53,100.33 IC19.17
  Bottom 0.305: IC28.7 IC26.14 | v91.44,90.17 92.08,89.53 127.64,89.53 128.91,90.81 133.99,90.81 v134.62,90.17 | IC19.17 142.24,100.33 143.51,101.6 151.76,101.6 160.66,110.49 IC20.33
PX6  (via drill 0.5)
  Top 0.305: IC28.8 90.81,101.6 92.08,100.33 92.08,93.98 90.17,92.08 v90.17,89.53 | IC19.18 136.53,102.87 133.99,100.33 133.99,91.44 133.35,90.81 v133.35,89.53
  Bottom 0.305: IC26.13 IC28.8 | v90.17,89.53 90.81,88.9 128.27,88.9 129.54,90.17 132.72,90.17 v133.35,89.53 | IC19.18 142.24,102.87 143.51,104.14 151.76,104.14 160.66,113.03 IC20.34
PX7  (via drill 0.5)
  Top 0.305: IC28.9 89.53,99.06 88.27,97.79 88.27,93.98 86.36,92.08 v86.36,90.81 | v132.08,88.9 132.08,90.81 133.35,92.08 133.35,102.23 136.53,105.41 IC19.19
  Bottom 0.305: IC28.9 IC26.12 | v86.36,90.81 88.27,88.27 128.91,88.27 130.18,89.53 131.44,89.53 v132.08,88.9 | IC19.19 142.24,105.41 143.51,106.68 151.76,106.68 160.66,115.57 IC20.35
PY0  (via drill 0.5)
  Top 0.305: IC27.19 61.59,116.84 62.87,118.11 62.87,127 v65.41,129.54 | v133.35,124.46 132.72,123.83 132.72,109.22 132.08,108.58 v132.08,105.41
  Bottom 0.305: v65.41,129.54 66.04,130.18 117.47,130.18 120.65,127 123.19,127 126.36,123.83 132.72,123.83 v133.35,124.46 152.4,124.46 160.02,116.84 165.1,116.84 165.74,116.2 165.74,96.52 164.47,95.25 IC20.27 | IC19.10 v132.08,105.41
PY1  (via drill 0.5)
  Top 0.305: IC27.18 61.59,114.3 63.5,116.2 63.5,125.73 v66.67,128.91 | v119.38,125.73 118.75,125.09 118.75,121.28 120.02,120.02 120.02,109.22 121.28,107.95 IC19.9 123.19,107.95 123.83,107.31 123.83,102.87 127,99.69 127,88.27 125.73,87 125.73,85.09 130.18,80.64 v131.44,80.64
  Bottom 0.305: v66.67,128.91 67.31,129.54 117.16,129.54 119.38,127.32 v119.38,125.73 | IC20.26 164.47,92.71 165.74,91.44 165.74,79.38 164.47,78.11 142.88,78.11 140.34,80.64 v131.44,80.64
PY2  (via drill 0.5)
  Top 0.305: IC27.17 60.33,111.76 59.05,113.03 59.05,125.09 v64.14,130.18 | v132.72,87 132.08,87 130.81,88.27 130.81,109.86 v131.44,110.49 132.08,111.12 v132.08,125.09
  Bottom 0.305: v64.14,130.18 64.77,130.81 123.19,130.81 123.83,130.18 123.83,127.64 127,124.46 131.44,124.46 v132.08,125.09 | IC20.24 156.84,87.63 155.57,86.36 143.51,86.36 142.88,87 v132.72,87 | IC19.8 v131.44,110.49
PY3  (via drill 0.5)
  Top 0.305: IC27.16 60.33,109.22 58.42,111.12 58.42,126.36 v62.87,130.81 | v130.81,125.73 v130.81,113.03 130.18,112.39 130.18,87.63 132.08,85.72 v133.99,85.72
  Bottom 0.305: v62.87,130.81 63.5,131.44 123.83,131.44 124.46,130.81 124.46,128.27 127.64,125.09 130.18,125.09 v130.81,125.73 | IC20.23 156.84,85.09 155.57,83.82 143.51,83.82 141.6,85.72 v133.99,85.72 | IC19.7 v130.81,113.03
PY4  (via drill 0.5)
  Top 0.305: IC27.15 60.33,106.68 57.78,109.22 57.78,127.64 v61.59,131.44 | v129.54,126.36 v129.54,115.57 129.54,86.68 v131.44,84.77
  Bottom 0.305: v61.59,131.44 62.23,132.08 124.46,132.08 125.09,131.44 125.09,128.91 128.27,125.73 128.91,125.73 v129.54,126.36 | IC20.22 156.84,82.55 155.57,81.28 143.51,81.28 140.97,83.82 132.4,83.82 v131.44,84.77 | IC19.6 v129.54,115.57
PY5  (via drill 0.5)
  Top 0.305: IC27.14 60.33,104.14 57.15,107.31 57.15,128.91 v60.33,132.08 | v128.27,127.64 v128.27,118.11 128.27,114.3 128.91,113.67 128.91,85.72 v132.72,81.92
  Bottom 0.305: v60.33,132.08 60.96,132.72 125.09,132.72 125.73,132.08 125.73,129.54 127.64,127.64 v128.27,127.64 | IC20.21 156.84,80.01 155.57,78.74 143.51,78.74 140.34,81.92 v132.72,81.92 | IC19.5 v128.27,118.11
PY6  (via drill 0.5)
  Top 0.305: IC27.13 60.33,101.6 56.52,105.41 56.52,130.18 v59.05,132.72 | v127.64,129.54 127,128.91 v127,120.65 127,113.67 128.27,112.39 128.27,84.45 v129.54,83.19
  Bottom 0.305: v59.05,132.72 59.69,133.35 125.73,133.35 126.36,132.72 126.36,130.81 v127.64,129.54 | IC20.20 143.51,80.01 140.34,83.19 v129.54,83.19 | IC19.4 v127,120.65
PY7  (via drill 0.5)
  Top 0.305: IC27.12 60.33,99.06 55.88,103.5 55.88,131.44 v57.78,133.35 | IC19.3 124.46,123.19 | 124.46,123.19 124.46,128.91 v127.64,133.35 | 124.46,123.19 124.46,103.5 127.64,100.33 127.64,87 v127,86.36
  Bottom 0.305: v57.78,133.35 58.42,133.99 127,133.99 v127.64,133.35 | IC20.19 143.51,82.55 141.6,84.45 133.35,84.45 131.44,86.36 v127,86.36
PZ0  (via drill 0.5)
  Top 0.305: IC25.19 73.66,116.84 74.93,118.11 74.93,121.92 v76.83,123.83 | IC19.25 136.53,120.65 135.25,119.38 v135.25,114.3
  Bottom 0.305: v76.83,123.83 77.47,124.46 111.12,124.46 114.3,121.28 114.3,115.57 115.57,114.3 v135.25,114.3 | IC19.25 140.34,120.65 145.41,115.57 IC20.6
PZ1  (via drill 0.5)
  Top 0.305: IC25.18 72.39,114.3 71.12,115.57 71.12,120.02 v75.56,124.46
  Bottom 0.305: v75.56,124.46 76.2,125.09 111.76,125.09 114.94,121.92 114.94,118.11 116.2,116.84 135.25,116.84 136.53,118.11 IC19.24 140.34,118.11 145.41,113.03 IC20.7
PZ2  (via drill 0.5)
  Top 0.305: IC25.17 72.39,111.76 70.48,113.67 70.48,121.28 v74.3,125.09 | v116.2,118.75 v116.2,109.22
  Bottom 0.305: v74.3,125.09 74.93,125.73 112.39,125.73 115.57,122.56 115.57,119.38 v116.2,118.75 | IC20.8 IC19.21 136.53,110.49 135.25,109.22 v116.2,109.22
PZ3  (via drill 0.5)
  Top 0.305: IC25.16 72.39,109.22 69.85,111.76 69.85,122.56 v73.03,125.73 | IC19.23 139.06,115.57 | 139.06,115.57 140.34,115.57 147.96,107.95 IC20.9 | v139.06,119.38 139.06,115.57
  Bottom 0.305: v73.03,125.73 73.66,126.36 113.03,126.36 116.2,123.19 116.2,120.65 117.47,119.38 v139.06,119.38
PZ4  (via drill 0.5)
  Top 0.305: IC25.15 72.39,106.68 69.22,109.86 69.22,123.83 v71.75,126.36 | IC19.2 121.28,125.73 120.02,124.46 v120.02,121.92
  Bottom 0.305: v71.75,126.36 72.39,127 113.35,127 116.84,123.51 116.84,122.56 117.47,121.92 v120.02,121.92
PZ5  (via drill 0.5)
  Top 0.305: IC25.14 72.39,104.14 68.58,107.95 68.58,125.09 v70.48,127
  Bottom 0.305: v70.48,127 71.12,127.64 113.67,127.64 116.84,124.46 123.83,124.46 125.09,123.19 IC19.26
PZ6  (via drill 0.5)
  Top 0.305: IC25.13 72.39,101.6 67.94,106.05 67.94,126.36 v69.22,127.64 | v116.2,126.68 116.52,126.68 127,137.16 v127.64,137.16 | IC3.1 v142.24,137.16
  Bottom 0.305: v69.22,127.64 69.85,128.27 114.62,128.27 v116.2,126.68 | v127.64,137.16 v142.24,137.16
PZ7  (via drill 0.5)
  Top 0.305: IC25.12 72.39,99.06 67.31,104.14 67.31,127.64 v67.94,128.27 | v116.2,128.27 126.36,138.43 v128.91,138.43 | IC3.2 v144.78,138.43
  Bottom 0.305: v67.94,128.27 68.58,128.91 115.57,128.91 v116.2,128.27 | v144.78,138.43 v128.91,138.43
R/!W  (via drill 0.5)
  Top 0.305: 37.47,72.39 34.92,69.85 34.92,44.45 v37.47,41.91 | IC29.1 77.47,40.64 78.11,40.01 78.11,39.37 75.56,36.83 v75.56,30.48 | v130.81,64.77 v130.81,27.94 | IC1.11 37.47,72.39 | 37.47,72.39 v37.47,88.9
  Bottom 0.305: IC40.29 122.56,64.77 123.83,66.04 129.54,66.04 v130.81,64.77 132.72,64.77 133.99,63.5 141.6,63.5 142.88,64.77 IC15.1 | v37.47,41.91 46.99,41.91 48.26,43.18 52.7,43.18 60.33,35.56 67.94,35.56 73.03,30.48 v75.56,30.48 88.9,30.48 90.17,29.21 IC33.4 96.52,29.21 97.79,27.94 v130.81,27.94 | IC34.22 v37.47,88.9
RAM  (via drill 0.5)
  Top 0.305: IC40.24 121.92,52.07 123.19,50.8 123.19,46.99 | 123.19,46.99 IC40.22 | 123.19,46.99 v123.19,26.67
  Bottom 0.305: IC33.20 v123.19,26.67
RES  (via drill 0.5)
  Top 0.305: IC24.1 102.23,121.28 v99.06,121.28 | IC34.34 47.62,119.38 46.35,118.11 46.35,85.72 47.62,84.45 47.62,40.64 48.9,39.37 IC12.14
  Top 0.61: C43.+ 45.72,36.83 R41.2 48.26,39.37 IC12.14
  Bottom 0.305: IC34.34 48.9,119.38 52.07,122.56 97.79,122.56 v99.06,121.28 | R40.2 IC12.14
  Bottom 0.61: R39.1 43.18,28.57 C43.+
ROM  (via drill 0.5)
  Top 0.305: IC43.22 139.7,52.07 138.43,50.8 138.43,46.99 | 138.43,46.99 IC43.20 | 138.43,46.99 138.43,29.84 v137.79,29.21
  Bottom 0.305: IC33.21 v137.79,29.21
RPIO  (via drill 0.5)
  Top 0.305: IC10.1 96.52,132.72 107.31,121.92 v107.31,83.19
  Bottom 0.305: IC10.19 92.08,139.7 93.34,140.97 97.79,140.97 98.42,140.34 98.42,138.43 97.16,137.16 IC10.1 | v107.31,83.19 121.92,83.19 131.44,73.66 154.31,73.66 157.48,70.48 157.48,54.61 152.4,49.53 IC15.18
RST
  Bottom 0.305: R40.1 34.92,38.1 26.04,38.1 24.77,39.37 J8.14
RXD1
  Bottom 0.305: IC2.13 58.42,154.94 55.88,152.4 P5.4
RXD2
  Bottom 0.305: IC2.4 67.94,144.78 66.67,146.05 45.72,146.05 45.09,146.69 44.45,147.32 43.18,148.59 40.64,148.59 40.01,149.22 40.01,151.13 41.27,152.4 P4.4
TA0
  Bottom 0.305: IC12.6 48.26,59.69 46.99,58.42 26.04,58.42 24.77,59.69 J8.6
TA1
  Bottom 0.305: J8.7 24.77,57.15 26.04,55.88 46.99,55.88 48.26,57.15 IC12.7
TA2
  Bottom 0.305: IC12.8 48.26,54.61 46.99,53.34 26.04,53.34 24.77,54.61 J8.8
TA3
  Bottom 0.305: J8.9 24.77,52.07 26.04,50.8 46.99,50.8 48.26,52.07 IC12.9
TA4
  Bottom 0.305: J8.10 24.77,49.53 26.04,48.26 46.99,48.26 48.26,49.53 IC12.10
TA5
  Bottom 0.305: J8.16 24.13,34.29 25.4,33.02 46.99,33.02 48.26,34.29 IC12.16
TA6
  Bottom 0.305: IC12.15 48.26,36.83 46.99,35.56 25.4,35.56 24.13,36.83 J8.15
TA7
  Bottom 0.305: IC12.11 48.26,46.99 46.99,45.72 26.04,45.72 24.77,46.99 J8.11
TB0
  Bottom 0.305: J8.3 24.77,67.31 26.04,66.04 34.92,66.04 36.2,67.31 IC1.13
TB1
  Bottom 0.305: IC1.14 36.83,63.5 26.04,63.5 24.77,64.77 J8.4
TB2
  Bottom 0.305: J8.5 24.77,62.23 26.04,60.96 35.56,60.96 36.83,62.23 IC1.15
TB3  (via drill 0.5)
  Top 0.305: v36.83,66.04 39.37,66.04 40.01,65.41 40.01,55.88 38.73,54.61 IC1.18
  Bottom 0.305: J8.37 35.56,64.77 v36.83,66.04
TB4  (via drill 0.5)
  Top 0.305: IC8.3 8.89,129.54 6.35,127 6.35,109.54 v6.03,109.22 5.71,108.9 5.71,78.74 v15.88,68.58
  Bottom 0.305: J8.38 26.04,67.31 24.77,68.58 v15.88,68.58 | IC7.2 v6.03,109.22
TB5  (via drill 0.5)
  Top 0.305: IC8.6 8.89,121.92 7.62,120.65 7.62,111.12 v8.26,110.49 7.62,109.86 7.62,81.92 17.14,72.39 J8.1
  Bottom 0.305: IC7.15 13.97,109.22 12.7,110.49 v8.26,110.49
TB6  (via drill 0.5)
  Top 0.305: IC8.4 8.89,127 6.99,125.09 6.99,96.84 v6.67,96.52 6.99,96.2 6.99,80.01 v15.88,71.12
  Bottom 0.305: J8.39 26.04,69.85 24.77,71.12 v15.88,71.12 | v6.67,96.52 IC7.7
TB7  (via drill 0.5)
  Top 0.305: v20.95,125.73 20.95,96.52 | 20.95,96.52 20.95,72.39 18.41,69.85 J8.2 | IC7.10 20.95,96.52
  Bottom 0.305: IC8.5 10.79,124.46 14.61,128.27 18.41,128.27 v20.95,125.73
TXD1  (via drill 0.5)
  Top 0.305: IC2.3 69.85,142.24 66.67,145.41 v66.67,156.21 | R2.2 55.24,157.48 52.7,154.94 P5.5
  Bottom 0.305: v66.67,156.21 57.15,156.21 55.88,154.94 P5.5
TXD2
  Top 0.305: R1.2 45.09,157.48 42.55,154.94 P4.5
  Bottom 0.305: IC2.12 57.15,157.48 55.88,156.21 43.81,156.21 42.55,154.94 P4.5
VCC  (via drill 0.5)  (1 unrouted)
  Top 0.305: IC30.2 IC30.15 | IC11.11 106.05,144.78 | IC20.12 IC20.13 147.96,97.79 146.69,96.52 146.69,93.98 147.96,92.71 IC20.15 IC20.16 | IC11.13 IC11.14 | 164.47,149.86 166.37,147.96 IC4.1 | R15.2 132.08,157.48
  Top 0.61: R3.1 192.41,76.2
  Top 1.27: IC40.32 122.56,72.39 125.09,69.85 125.09,69.22 | 125.09,69.22 IC43.1 | 40.64,36.83 P1.2 | 71.12,41.91 72.39,43.18 72.39,67.31 C10.1 JP1.3 IC30.15 IC30.16 | 71.12,41.91 C18.1 66.04,34.29 IC12.25 64.14,34.29 59.69,29.84 C1.1 59.69,12.7 QG2.14 64.77,3.17 | IC29.20 71.12,41.91 | C7.1 92.08,65.41 92.71,64.77 92.08,64.77 90.81,63.5 90.81,40.64 C5.1 | IC13.20 84.45,36.83 83.19,35.56 83.19,12.7 C8.1 84.45,3.17 | 99.69,8.89 98.42,10.16 98.42,33.02 99.69,34.29 IC33.23 IC33.24 C11.1 | 99.69,8.89 IC33.13 IC33.14 | 99.69,8.89 C6.1 99.69,3.17 | 15.88,134.62 C16.1 13.34,140.97 3.17,140.97 | 15.88,134.62 IC8.14 | 15.88,134.62 14.61,133.35 14.61,115.57 | 14.61,115.57 14.61,111.76 | 14.61,111.76 C13.+ | 14.61,111.76 IC7.16 | 14.61,115.57 C20.1 | 41.27,49.53 41.27,73.03 C9.1 v39.37,92.71 39.37,135.89 40.01,136.53 C17.1 41.91,140.34 P4.1 | 41.27,49.53 IC1.20 | 41.27,49.53 41.27,43.81 40.64,43.18 40.64,36.83 | IC40.1 109.22,75.56 109.22,117.47 111.12,119.38 IC24.20 111.76,121.28 103.5,129.54 IC11.14 104.78,137.16 106.05,138.43 106.05,144.78 106.05,154.31 C23.1 106.68,157.48 | 106.68,157.48 SWAP.A PGM.A EXTRA.A DATA.A 132.08,157.48 132.72,157.48 | IC10.20 88.9,131.44 85.72,128.27 IC26.20 | 161.93,67.31 C21.1 148.59,69.22 142.24,69.22 IC43.28 | C25.1 111.12,3.17 | 40.01,3.17 C24.1 40.64,7.62 40.64,36.83 | C3.+ 3.17,71.12 | R2.1 55.24,164.47 | 132.72,157.48 132.72,164.47 | 106.68,157.48 106.68,164.47 | IC19.28 137.16,151.13 | 137.16,151.13 137.16,153.67 | 137.16,153.67 132.72,157.48 | 137.16,151.13 C15.1 141.6,151.13 | 141.6,151.13 142.24,151.76 IC3.16 | 141.6,151.13 142.88,149.86 163.19,149.86 | 163.19,149.86 164.47,149.86 166.37,151.76 IC4.14
  Top 1.27: 163.19,149.86 C30.1 163.19,164.47 | X1.1 124.46,10.16 | C14.+ 144.78,19.68 147.32,17.14 147.32,3.17 | IC20.25 165.1,90.17 167,88.27 167,76.83 161.93,71.75 161.93,67.31 | IC20.16 146.05,90.17 125.09,69.22 | C4.+ 137.16,153.67 | R43.1 38.73,164.47 | R1.1 45.09,164.47 | R44.1 57.78,164.47 | 164.47,41.27 164.47,57.15 161.93,59.69 161.93,67.31 | PWR.A 12.7,164.47 | 164.47,41.27 160.02,41.27 156.21,37.47 P3.1 | P4.1 40.64,144.78 36.83,148.59 36.83,164.47 | 59.69,144.78 P5.1 P4.1 | 59.69,144.78 59.69,164.47 | IC2.20 62.23,137.16 59.69,139.7 59.69,144.78 | JP7.2 162.56,7.62 164.47,9.53 164.47,20.32 | 164.47,20.32 164.47,41.27 | 164.47,20.32 168.91,20.32
  Top 2.54: 124.46,3.17 111.12,3.17 99.69,3.17 84.45,3.17 64.77,3.17 40.01,3.17 26.04,3.17 3.17,26.04 3.17,71.12 3.17,140.97 3.17,157.48 10.16,164.47 12.7,164.47 36.83,164.47 38.73,164.47 45.09,164.47 55.24,164.47 57.78,164.47 59.69,164.47 106.68,164.47 132.72,164.47 163.19,164.47 179.07,164.47 192.41,151.13 192.41,76.2 192.41,4.45 191.13,3.17 173.35,3.17 | 124.46,3.17 147.32,3.17 162.56,3.17 | 162.56,3.17 173.35,3.17 | 173.35,3.17 173.35,15.88 SX5.3 | 124.46,10.16 124.46,3.17 | 162.56,3.17 JP7.2
  Bottom 0.305: IC30.2 IC30.3 68.58,92.08 67.31,93.34 64.77,93.34 63.5,92.08 IC30.5 | IC30.11 60.96,84.45 62.23,85.72 69.85,85.72 71.12,84.45 IC30.15 | IC34.24 40.64,93.98 v39.37,92.71 IC34.20 | IC4.1 166.37,144.15 167.64,142.88 171.45,142.88 | 171.45,142.88 175.26,142.88 176.53,144.15 IC4.5 | IC4.3 171.45,142.88
  Bottom 0.61: IC20.16 IC20.25 | P1.2 43.18,36.83 R41.1
  Bottom 1.27: IC40.30 IC43.1 IC43.28 | IC27.20 60.96,121.28 73.03,121.28 | 73.03,121.28 IC25.20 | 73.03,121.28 85.72,121.28 | 85.72,121.28 IC26.20 | 85.72,121.28 95.89,121.28 IC28.20 R38.1 102.87,121.28 111.76,121.28 IC24.20 | IC13.20 89.53,36.83 C5.1 93.98,39.37 96.52,36.83 IC33.24 | IC40.32 116.2,72.39 | 116.2,72.39 IC40.1 IC40.2 104.78,69.85 103.5,68.58 C7.1 90.17,66.67 73.03,66.67 C10.1 | C2.1 116.2,72.39 | 77.47,135.25 65.41,135.25 IC2.20 62.23,137.16 60.33,139.06 C17.1 41.27,140.97 36.2,140.97 33.66,138.43 C16.1 | 77.47,135.25 IC9.20 | 77.47,135.25 88.9,135.25 | 88.9,135.25 IC10.20 | 88.9,135.25 100.33,135.25 | 100.33,135.25 101.6,135.25 IC11.14 | IC7.16 IC7.1 | C19.1 100.33,135.25 | C21.1 150.5,64.77 | 150.5,64.77 IC15.24 | 150.5,64.77 146.69,60.96 146.69,40.64 150.5,36.83 | 150.5,36.83 IC15.13 P3.1 | 150.5,36.83 C22.1 144.78,28.57 C14.+ | C13.+ 14.61,86.36 | 14.61,86.36 14.61,76.83 C3.+ | IC34.20 14.61,86.36
WPIO  (via drill 0.5)
  Top 0.305: IC9.11 81.92,160.02 83.82,161.93 90.81,161.93 91.44,161.29 91.44,134.62 106.05,120.65 v106.05,81.92
  Bottom 0.305: v106.05,81.92 121.92,81.92 130.81,73.03 153.67,73.03 156.84,69.85 156.84,56.52 152.4,52.07 IC15.19
X2
  Bottom 0.305: IC12.17 48.9,31.75 47.62,30.48 47.62,24.77 45.09,22.23 37.47,22.23 35.56,20.32 P2.2
X2S
  Bottom 0.305: P7.3 66.04,13.97 58.42,6.35 48.26,6.35 44.45,10.16 34.29,10.16 33.02,11.43 P2.1 33.02,17.14 18.41,31.75 J8.17

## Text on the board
tNames: 12V | 21V | 5V | GND | TxD | EVM7000-3 | RxD | DTR | Ruud Baltissen | DSR | Credits: / Jaak Bartok / Fred Jan Kraan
